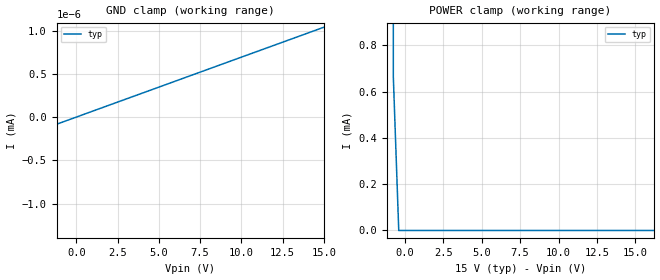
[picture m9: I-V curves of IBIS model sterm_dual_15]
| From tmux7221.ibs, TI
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| sterm_dual_15
[Model]   sterm_dual_15
Model_type   Terminator
|   typ   min   max
C_comp   1.598234e-11   NA   NA
[Voltage Range]   15   NA   NA
[Temperature Range]   27   NA   NA
[Power Clamp Reference]   15   NA   NA
[GND Clamp Reference]   0   NA   NA
[GND Clamp]
|   Voltage   I(typ)   I(min)   I(max)
-20V      -3.998A    NA         NA
-15.4V    -5.116nA   NA         NA
-15.05V   -1.042nA   NA         NA
15V       1.038nA    NA         NA
[POWER Clamp]
|   Voltage   I(typ)   I(min)   I(max)
-5V       4.766A     NA         NA
-1.111V   115.3mA    NA         NA
-757.6mV  664.9uA    NA         NA
-404mV    3.734nA    NA         NA
30V       -1.038nA   NA         NA
